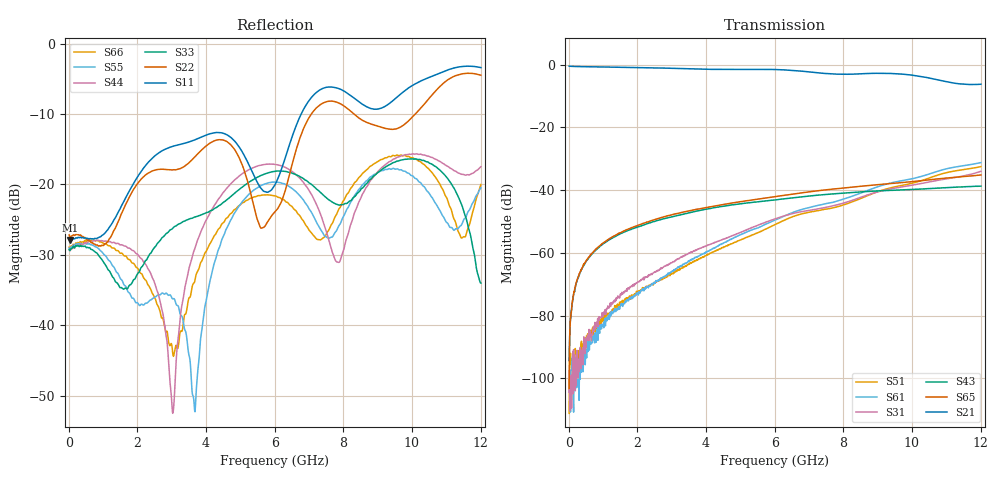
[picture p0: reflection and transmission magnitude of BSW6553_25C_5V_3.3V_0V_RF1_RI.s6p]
! Agilent Technologies	N5230C	MY49001333	A.09.33.09
!	Test time	=	2026-05-26 10:00
!	Product	=	BSW6553
!	Temp	=	25C
!	Logic	=	RF1
!	Port1	=	RFC
!	Port2	=	RF1
!	Port3	=	RF2
!	Port4	=	RF3
!	Port5	=	RF4
!	Port6	=	RF5
!S6P File: Measurements: <S11,S12,S13,S14,S15,S16>,
!<S21,S22,S23,S24,S25,S26>,
!<S31,S32,S33,S34,S35,S36>,
!<S41,S42,S43,S44,S45,S46>,
!<S51,S52,S53,S54,S55,S56>,
!<S61,S62,S63,S64,S65,S66>;
# HZ S RI R 50
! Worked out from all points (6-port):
!   1201 points, 10 MHz to 12.01 GHz, reference 50 ohm
!   strongest paths, dB at 10 MHz, 3.01 GHz, 6.01 GHz, 9.01 GHz, 12.01 GHz:
!     S21: -0.5, -1.2, -1.6, -2.8, -6.3
!     S65: -103.2, -47.8, -42.1, -38.3, -35.2
!     S43: -94.3, -48.5, -43.1, -40.3, -38.7
!     S31: -104.4, -63.1, -49.2, -40.6, -34.0
!     S61: -99.9, -65.8, -49.5, -38.9, -31.3
!     S51: -111.1, -66.6, -51.0, -40.5, -32.5
!   lowest |S11| = -27.9 dB at 40 MHz (marker M1), VSWR 1.08, Z = 54.2 - j0.518 ohm
!   |S11| at or under -10 dB: start of sweep to 6.774 GHz
